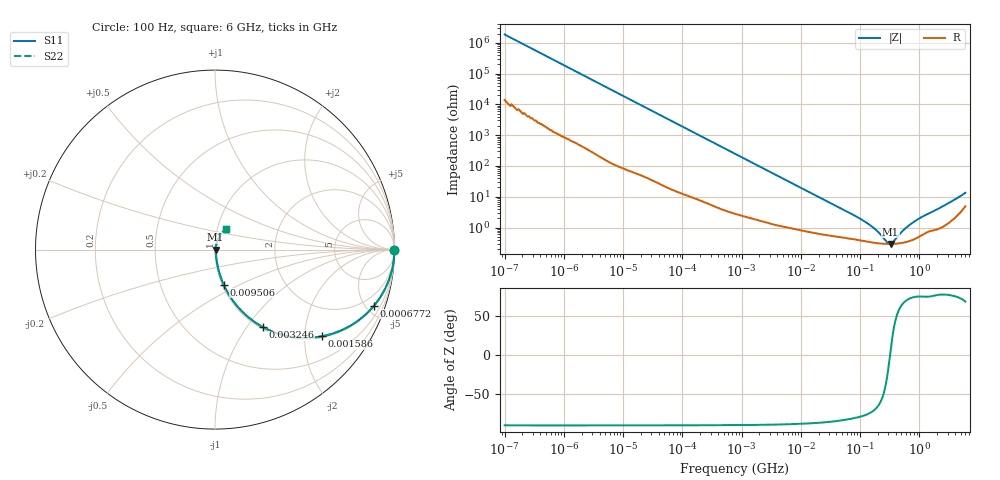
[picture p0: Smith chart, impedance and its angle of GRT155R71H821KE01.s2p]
!Murata Part Number: GRT155R71H821KE01
!These Parameters are Measured in Series Mode Connection
!Data Generated on Jun 19, 2026
!  o--ll--o
!Port1  Port2
!  o------o
!Operation Temp=25[degC], DC Bias Voltage=0[V]
!Freq. Start=100[Hz] Stop=6[GHz] 401[Steps]
# Hz S RI R 50
!Freq.(Hz) S11(Real) S11(Imag) S21(Real) S21(Imag) S12(Real) S12(Imag) S22(Real) S22(Imag)
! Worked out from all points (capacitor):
!   401 points, 100 Hz to 6 GHz, reference 50 ohm
!   read as one part in series: C = 852 pF near 109 Hz
!   lowest |Z| = 295 mohm at 326.7 MHz (marker M1)
!   series resonance near 320.4 MHz, so ESL is about 290 pH
!   S11 on the Smith chart (normalised r, x): 100 Hz: open; 677.2 kHz: 1.06, -5.67; 1.586 MHz: 1.04, -2.43; 3.246 MHz: 1.03, -1.20; 9.506 MHz: 1.02, -0.41; 6 GHz: 1.10, +0.25
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100  1 -5.36e-05  4e-07 5.36e-05  4e-07 5.36e-05  1 -5.36e-05
196  1 -0.000105  6e-07 0.000105  6e-07 0.000105  1 -0.000105
2008  1 -0.00107  6.1e-06 0.00107  6.1e-06 0.00107  1 -0.00107
40335  0.9994 -0.0212  0.000572 0.0212  0.000572 0.0212  0.9994 -0.0212
202169  0.9881 -0.1046  0.0119 0.1046  0.0119 0.1046  0.9881 -0.1046
677235  0.8867 -0.3116  0.1133 0.3116  0.1133 0.3116  0.8867 -0.3116
774597  0.8574 -0.3441  0.1426 0.3441  0.1426 0.3441  0.8574 -0.3441
1585629  0.5956 -0.4831  0.4044 0.4831  0.4044 0.4831  0.5956 -0.4831
2268635  0.4227 -0.4849  0.5773 0.4849  0.5773 0.4849  0.4227 -0.4849
3245845  0.2679 -0.4322  0.7321 0.4322  0.7321 0.4322  0.2679 -0.4322
5311619  0.1257 -0.3176  0.8743 0.3176  0.8743 0.3176  0.1257 -0.3176
9506416  0.0482 -0.195  0.9518 0.195  0.9518 0.195  0.0482 -0.195
1.555665e7  0.0224 -0.1235  0.9776 0.1235  0.9776 0.1235  0.0224 -0.1235
1.220122e8  0.00378 -0.0149  0.9962 0.0149  0.9962 0.0149  0.00378 -0.0149
1.825626e8  0.0032 -0.00799  0.9968 0.00799  0.9968 0.00799  0.0032 -0.00799
2.856706e8  0.00294 -0.00157  0.9971 0.00157  0.9971 0.00157  0.00294 -0.00157
3.124326e8  0.00293 -0.000342  0.9971 0.000342  0.9971 0.000342  0.00293 -0.000342
3.267395e8  0.00293 0.000271  0.9971 -0.000271  0.9971 -0.000271  0.00293 0.000271
3.737127e8  0.00296 0.00212  0.997 -0.00212  0.997 -0.00212  0.00296 0.00212
5.59173e8  0.00333 0.00806  0.9967 -0.00806  0.9967 -0.00806  0.00333 0.00806
8.366708e8  0.00446 0.0152  0.9955 -0.0152  0.9955 -0.0152  0.00446 0.0152
6e9  0.0604 0.1126  0.9396 -0.1126  0.9396 -0.1126  0.0604 0.1126
